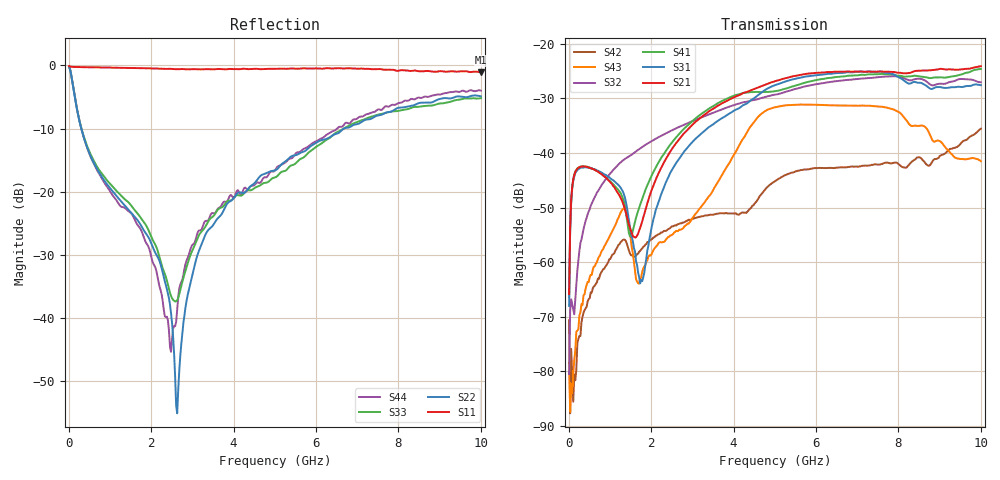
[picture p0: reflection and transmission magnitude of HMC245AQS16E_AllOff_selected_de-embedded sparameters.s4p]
! Device:	HMC245AQS16E
! Description:	GaAs MMIC SP3T Non-Reflective Switch
! Package:	LP3E - 16 pin 3x3mm QFN plastic package
! Frequency:	DC -  3.5 GHz
! Ports:
! RFC = Port 1
! RF1 = Port 2
! RF2 = Port 3
! RF3 = Port 4
! State: All Off
! Supply Voltage:
! Vdd = 5 V
! Control Voltages:
! VA  = 5 V
! VB  = 5 V
! Data:	Data was collected using a calibrated network analyzer with AFR software.
!	Fixtures were calculated using AFR and fixturing was applied to collect
!	this Deembedded  S Parameter data of HMC245AQS16E
! Note:	Analog Devices supplies this data as a sample of measured data at the package pin
!	for this product.  Your particular data for this product may vary.
!	Data was taken at 25 degrees C.
!	Analog Devices reserves the right to change this data at anytime.
# GHz S  dB  R 50
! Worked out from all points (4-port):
!   401 points, 10 MHz to 10 GHz, reference 50 ohm
!   strongest paths, dB at 10 MHz, 2.507 GHz, 5.005 GHz, 7.503 GHz, 10 GHz:
!     S21: -65.8, -39.3, -26.9, -25.1, -24.1
!     S31: -68.0, -43.1, -27.6, -25.2, -27.6
!     S41: -66.4, -38.1, -28.7, -25.6, -24.7
!     S32: -80.5, -35.9, -29.4, -26.2, -27.1
!     S43: -78.4, -55.0, -31.7, -31.5, -41.5
!     S42: -70.6, -53.4, -45.2, -42.2, -35.6
!   lowest |S11| = -1.1 dB at 10 GHz (marker M1), VSWR 15.97, Z = 47 - j182 ohm
!   |S11| at or under -10 dB: nowhere
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0.01  -0.11 -0.8  -67.65 87.0  -69.14 80.1  -68.04 99.6
      -65.84 94.2  -0.18 -5.8  -81.19 -106.2  -78.91 -4.7
      -68.00 84.9  -80.49 -35.8  -0.18 -5.7  -79.02 -66.9
      -66.42 120.9  -70.63 -72.2  -78.39 -27.2  -0.18 -5.8
0.6094  -0.29 -29.4  -43.04 -0.7  -42.98 -4.9  -43.00 -3.3
        -43.03 -0.5  -15.46 -70.5  -48.40 98.2  -64.50 98.9
        -42.99 -4.9  -48.43 98.6  -15.10 -70.9  -60.86 96.3
        -42.97 -3.3  -64.44 97.2  -60.82 98.0  -15.55 -71.6
1.75825  -0.43 -88.2  -53.19 72.5  -63.63 25.9  -49.04 114.9
         -53.15 72.5  -25.40 -63.2  -39.09 85.9  -57.68 73.4
         -63.27 30.0  -39.07 86.0  -24.25 -69.0  -62.54 67.3
         -48.98 115.1  -57.69 73.0  -62.80 66.8  -26.13 -70.9
2.632375  -0.59 -139.8  -37.97 88.0  -41.55 90.5  -36.93 87.6
          -37.99 88.1  -55.15 60.8  -35.43 77.4  -53.04 64.3
          -41.58 90.6  -35.41 77.4  -37.21 -159.4  -54.27 94.6
          -36.93 87.6  -53.11 64.6  -54.32 93.7  -38.72 133.3
3.3067  -0.59 -179.9  -32.96 68.9  -35.89 70.1  -32.40 61.7
        -32.96 68.9  -26.97 108.7  -33.25 69.1  -51.42 56.0
        -35.90 70.2  -33.25 69.1  -25.66 141.2  -48.92 115.8
        -32.41 61.6  -51.47 55.9  -48.97 115.9  -24.69 116.7
5.179825  -0.50 94.0  -26.49 18.7  -27.13 14.0  -28.41 0.3
          -26.49 18.7  -15.57 79.7  -29.02 43.3  -44.35 51.3
          -27.13 14.0  -29.03 43.2  -16.83 103.6  -31.39 42.2
          -28.41 0.3  -44.37 51.3  -31.40 42.2  -15.67 87.1
10  -1.09 -29.0  -24.14 -73.4  -27.61 -118.2  -24.65 -123.0
    -24.14 -73.4  -4.90 -10.6  -27.05 -53.1  -35.59 21.6
    -27.61 -118.2  -27.07 -53.2  -5.18 -1.7  -41.49 -152.9
    -24.66 -123.0  -35.59 21.6  -41.52 -152.5  -4.00 -14.7
